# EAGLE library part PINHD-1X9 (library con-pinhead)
PIN HEADER
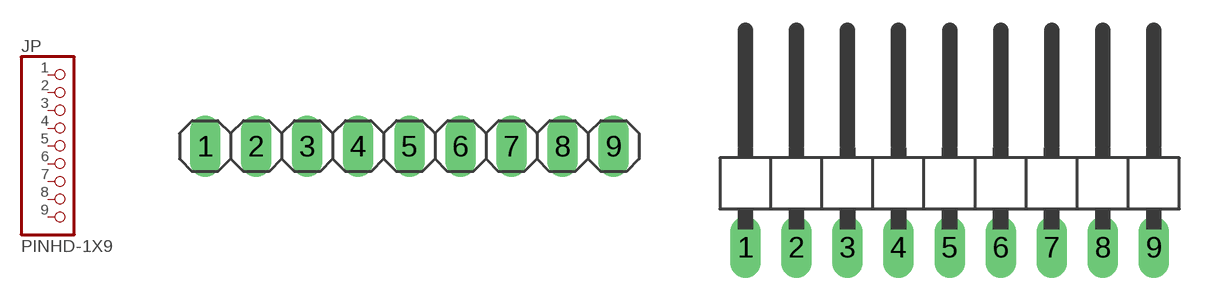
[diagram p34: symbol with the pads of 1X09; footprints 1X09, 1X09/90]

Designator prefix JP

## PINHD-1X9_2.54  [1X09]
1  1  pas
2  2  pas
3  3  pas
4  4  pas
5  5  pas
6  6  pas
7  7  pas
8  8  pas
9  9  pas

## PINHD-1X9_2.54-90°  [1X09/90]
Pads as for 1X09

## PINHD-1X9_2.00  [1X09M]
Pads as for 1X09

## PINHD-1X9_2.54-SMD  [1X09SMD]
Pads as for 1X09

## PINHD-1X9_2.54-SMD-90°  [1X09SMD/90]
Pads as for 1X09

## Footprint 1X09 (pad centres in mm)
PIN HEADER - 2.54
drill 1.016 long: 1 -10.16,0; 2 -7.62,0; 3 -5.08,0; 4 -2.54,0; 5 0,0; 6 2.54,0; 7 5.08,0; 8 7.62,0; 9 10.16,0

## Footprint 1X09/90 (pad centres in mm)
PIN HEADER - 2.54 90°
drill 1.016 long: 1 -10.16,-3.81; 2 -7.62,-3.81; 3 -5.08,-3.81; 4 -2.54,-3.81; 5 0,-3.81; 6 2.54,-3.81; 7 5.08,-3.81; 8 7.62,-3.81; 9 10.16,-3.81

## Footprint 1X09M (pad centres in mm)
PIN HEADER - 2
drill 0.914 square: 1 -8,0
drill 0.914: 2 -6,0; 3 -4,0; 4 -2,0; 5 0,0; 6 2,0; 7 4,0; 8 6,0; 9 8,0

## Footprint 1X09SMD (pad centres in mm)
PIN HEADER - 2.54 SMD
smd 1.016 x 3.302: 1 -1.27,1.27; 2 1.27,-1.27; 3 3.81,1.27; 4 6.35,-1.27; 5 8.89,1.27; 6 11.43,-1.27; 7 13.97,1.27; 8 16.51,-1.27; 9 19.05,1.27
